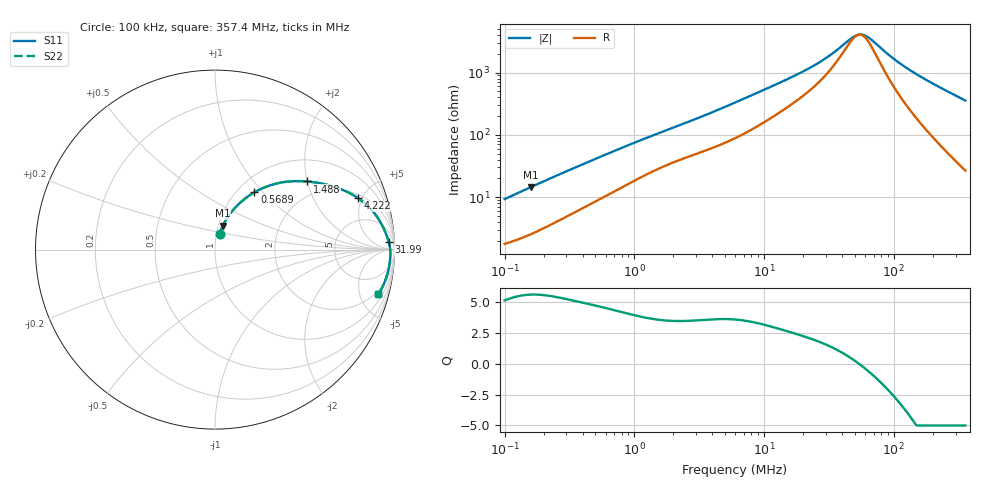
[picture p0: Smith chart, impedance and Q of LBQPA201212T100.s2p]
! LBQPA201212T100  S-PARAMETER MODEL  ( General Type )
! Model Generated by TAIYO YUDEN Corporation (http://www.ty-top.com)
! Version 1.0
! TAIYO YUDEN Control No. 191025NI43SB-FBB
! Copyright(c) 2019 TAIYO YUDEN CO.,LTD. All Rights Reserved.
! Product Description (link to TY-COMPAS)
! https://ds.yuden.co.jp/TYCOMPAS/or/detail?pn=LBQPA201212T100K&u=M
! Products Name : Inductors
! Characteristics :
!  Inductance : 10 uH , SRF(min) : 40 MHz , DC Resistance(max) : 1.56 Ohm
!  Rated Current : Saturation :240 mA , Temp Rise : 255 mA (20 degC)
!  Case Size : 2.0 x 1.25 / 0.079 x 0.049 [mm/inch] , Thickness : 1.25 / 0.049 [mm/inch]
!  (Conditions: Temperature = 25 degC , DC Bias Current/Voltage = 0A / 0V)
! External Node Assignments :
!  1  o---GGG---o  2
! GND o---------o GND
! Frequency Range : 0.1MHz  -  357.398349MHz  [ 402 STEP ]
# MHz S RI R 50
! Freq[MHz].  S11 Real  S11 Imag  S21 Real  S21 Imag  S12 Real  S12 Imag  S22 Real  S22 Imag
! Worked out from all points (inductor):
!   401 points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, 100 kHz to 357.4 MHz, reference 50 ohm
!   read as one part in series: L = 14.4 uH near 104.2 kHz
!   highest Q = 5.62 at 160.1 kHz (marker M1), where L = 14.3 uH
!   self-resonance near 54.08 MHz
!   S11 on the Smith chart (normalised r, x): 100 kHz: 1.04, +0.18; 568.9 kHz: 1.20, +0.90; 1.488 MHz: 1.55, +1.99; 4.222 MHz: 2.29, +4.66; 31.99 MHz: 22, +31; 357.4 MHz: 1.53, -7.09
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0.1  0.0253 0.0875  0.9747 -0.0875  0.9747 -0.0875  0.0253 0.0875
0.160069  0.0436 0.1338  0.9564 -0.1338  0.9564 -0.1338  0.0436 0.1338
0.25622  0.0811 0.1957  0.9189 -0.1957  0.9189 -0.1957  0.0811 0.1957
0.393689  0.1415 0.2622  0.8585 -0.2622  0.8585 -0.2622  0.1415 0.2622
0.568912  0.2197 0.3192  0.7803 -0.3192  0.7803 -0.3192  0.2197 0.3192
0.929467  0.3616 0.372  0.6384 -0.372  0.6384 -0.372  0.3616 0.372
1.487786  0.5127 0.3797  0.4873 -0.3797  0.4873 -0.3797  0.5127 0.3797
1.549909  0.5255 0.3785  0.4745 -0.3785  0.4745 -0.3785  0.5255 0.3785
2.532184  0.6704 0.3479  0.3296 -0.3479  0.3296 -0.3479  0.6704 0.3479
4.222477  0.7977 0.2866  0.2023 -0.2866  0.2023 -0.2866  0.7977 0.2866
6.101817  0.8646 0.2301  0.1354 -0.2301  0.1354 -0.2301  0.8646 0.2301
13.54851  0.9388 0.1201  0.0612 -0.1201  0.0612 -0.1201  0.9388 0.1201
23.53582  0.9607 0.0666  0.0393 -0.0666  0.0393 -0.0666  0.9607 0.0666
31.98693  0.9685 0.0414  0.0315 -0.0414  0.0315 -0.0414  0.9685 0.0414
48.15376  0.9749 0.00921  0.0251 -0.00921  0.0251 -0.00921  0.9749 0.00921
55.56615  0.9761 -0.00217  0.0239 0.00217  0.0239 0.00217  0.9761 -0.00217
64.11956  0.9769 -0.0138  0.0231 0.0138  0.0231 0.0138  0.9769 -0.0138
92.65788  0.9765 -0.0463  0.0235 0.0463  0.0235 0.0463  0.9765 -0.0463
120.8815  0.9738 -0.0735  0.0262 0.0735  0.0262 0.0735  0.9738 -0.0735
164.2869  0.9669 -0.1111  0.0331 0.1111  0.0331 0.1111  0.9669 -0.1111
247.3208  0.9473 -0.1753  0.0527 0.1753  0.0527 0.1753  0.9473 -0.1753
357.3983  0.9107 -0.2501  0.0893 0.2501  0.0893 0.2501  0.9107 -0.2501
